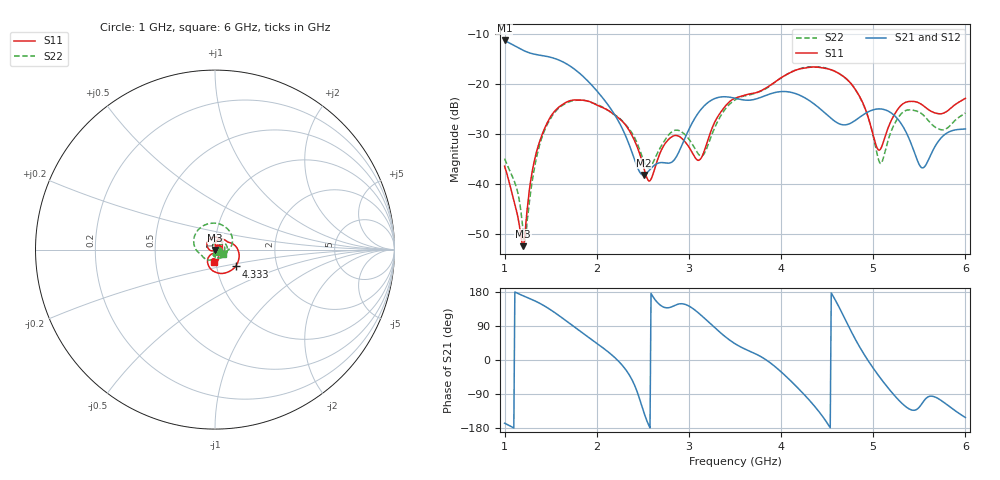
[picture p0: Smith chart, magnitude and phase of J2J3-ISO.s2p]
!Agilent Technologies,E8364B,MY43040528,A.07.50.67
!Agilent E8364B: A.07.50.67
!Date: Sunday, March 01, 2026 21:58:58
!Correction: S11(Full 2 Port(1,2))
!S21(Full 2 Port(1,2))
!S12(Full 2 Port(1,2))
!S22(Full 2 Port(1,2))
!S2P File: Measurements: S11, S21, S12, S22:
# Hz S  dB  R 50
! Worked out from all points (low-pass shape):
!   451 points, 1 GHz to 6 GHz, reference 50 ohm
!   highest |S21| = -11.30 dB at 1 GHz (marker M1); lowest = -38.1 dB at 2.511 GHz (marker M2)
!   |S21| within 3 dB of the highest: start of sweep to 1.403 GHz
!   lowest |S11| = -52.4 dB at 1.2 GHz (marker M3), VSWR 1.00, Z = 50.1 - j0.208 ohm
!   |S11| at or under -10 dB: start of sweep to end of sweep
!   |S22| runs from -51.3 to -16.6 dB; largest |S21 - S12| = 0.001
!   S11 on the Smith chart (normalised r, x): 1 GHz: 1.03, +0.01; 4.333 GHz: 1.23, -0.24; 6 GHz: 0.98, -0.14
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1e9  -36.40 19.2  -11.30 -166.8  -11.33 -166.7  -34.88 -29.7
1.133333e9  -45.64 3.5  -12.62 176.9  -12.65 176.9  -40.96 -40.7
1.2e9  -52.35 -59.4  -13.25 169.5  -13.29 169.5  -49.13 -70.7
1.233333e9  -47.29 -117.0  -13.53 166.1  -13.56 166.1  -49.94 -145.7
1.311111e9  -36.31 -151.6  -13.98 157.9  -14.02 158.0  -38.04 147.4
1.433333e9  -28.89 174.1  -14.39 142.5  -14.42 142.5  -29.25 104.3
1.844444e9  -23.22 83.5  -18.35 71.5  -18.37 71.5  -23.22 -5.7
2.288889e9  -27.66 20.8  -29.34 -17.5  -29.37 -17.5  -27.60 -87.7
2.511111e9  -36.73 10.6  -38.15 -138.2  -38.19 -138.1  -35.38 -104.1
2.577778e9  -39.29 44.8  -37.05 -179.2  -37.09 -179.1  -36.64 -82.7
2.666667e9  -34.73 72.3  -35.77 149.6  -35.81 149.6  -33.48 -63.9
2.866667e9  -30.27 50.6  -34.41 146.1  -34.45 146.2  -29.20 -95.3
3.122222e9  -35.03 70.1  -25.26 120.3  -25.30 120.3  -34.33 -108.4
3.5e9  -22.82 55.1  -22.83 43.0  -22.87 43.0  -23.18 -123.6
4.333333e9  -16.60 -39.3  -23.63 -113.4  -23.67 -113.3  -16.56 109.7
4.344444e9  -16.59 -41.0  -23.78 -116.5  -23.82 -116.5  -16.57 107.4
4.788889e9  -20.64 -114.1  -27.45 62.3  -27.49 62.3  -20.60 12.5
5.077778e9  -33.01 -88.4  -24.96 -47.7  -24.99 -47.6  -35.84 13.5
5.166667e9  -28.48 -61.4  -25.44 -75.3  -25.48 -75.3  -30.86 48.8
5.333333e9  -23.80 -77.5  -28.80 -119.2  -28.84 -119.2  -25.47 23.4
5.533333e9  -24.18 -101.0  -36.74 -113.4  -36.77 -113.3  -26.01 -15.4
6e9  -22.85 -94.8  -28.96 -151.8  -28.99 -151.8  -25.76 -29.2
